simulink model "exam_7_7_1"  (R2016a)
settings: Solver=VariableStepAuto  StartTime=0.0  StopTime=10.0  RelTol=1e-3

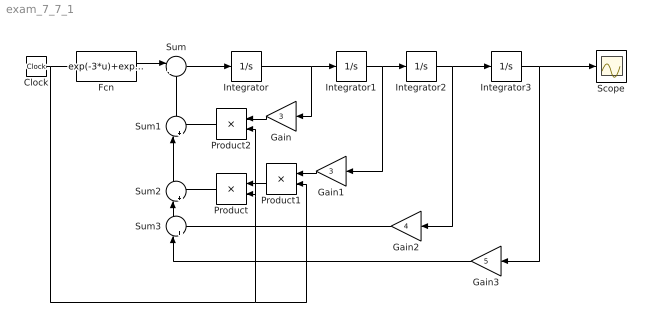
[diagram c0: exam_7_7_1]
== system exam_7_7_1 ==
  Clock : Clock
  Fcn : Fcn  Expr=exp(-3*u)+exp(-5*u)*sin(4*u+pi/3)
  Gain : Gain  Gain=3
  Gain1 : Gain  Gain=3
  Gain2 : Gain  Gain=4
  Gain3 : Gain  Gain=5
  Integrator : Integrator  InitialCondition=0.2
  Integrator1 : Integrator  InitialCondition=1/2
  Integrator2 : Integrator  InitialCondition=1/2
  Integrator3 : Integrator  InitialCondition=1
  Product : Product
  Product1 : Product
  Product2 : Product
  Scope : Scope
  Sum : Sum  Inputs=|+-
  Sum1 : Sum  Inputs=|++
  Sum2 : Sum  Inputs=|++
  Sum3 : Sum  Inputs=|++
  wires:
  Clock/1 -> Product2/2, Product/2, Product1/2, Fcn/1
  Fcn/1 -> Sum/1
  Sum/1 -> Integrator/1
  Integrator/1 -> Gain/1, Integrator1/1
  Integrator1/1 -> Gain1/1, Integrator2/1
  Integrator2/1 -> Gain2/1, Integrator3/1
  Integrator3/1 -> Gain3/1, Scope/1
  Gain2/1 -> Sum3/2
  Gain3/1 -> Sum3/1
  Sum1/1 -> Sum/2
  Sum2/1 -> Sum1/1
  Sum3/1 -> Sum2/1
  Gain1/1 -> Product1/1
  Product1/1 -> Product/1
  Product/1 -> Sum2/2
  Product2/1 -> Sum1/2
  Gain/1 -> Product2/1
